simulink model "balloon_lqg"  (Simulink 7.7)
settings: Solver=ode45  StartTime=0.0  StopTime=50000  RelTol=1e-3
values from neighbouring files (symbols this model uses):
  Akf = A_balloon - Kkf * C_balloon    [design_KF_balloon.m]
  Bkf = [B_balloon Kkf]    [design_KF_balloon.m]
  C = V*rho_a*c_a    [balloon_init.m]
  Ckf = eye(3)    [design_KF_balloon.m]
  Dkf = zeros(3,4)    [design_KF_balloon.m]
  f = f / 10    [balloon_init.m]
  g = 9.80665    [balloon_init.m]
  m = input('Inserire le prime due cifre (esclusi zeri) del proprio numero di matricola:\n\n')    [balloon_init.m]
  rho_a = 1.2928    [balloon_init.m]
  Ta = 20+273.15    (= 293.15)    [balloon_init.m]
  theta_t = theta_t/50    [balloon_init.m]
  V = V*m*2    [balloon_init.m]
  x1_0 = x1_d    [balloon_init.m]
  x2_0 = 100    [balloon_init.m]
  x2_d = 120    [balloon_init.m]
  x3_0 = 0    [balloon_init.m]
  x3_d = 0    [balloon_init.m]
undefined symbols (not defined in the file or in its folder): K
libraries: simulink x3

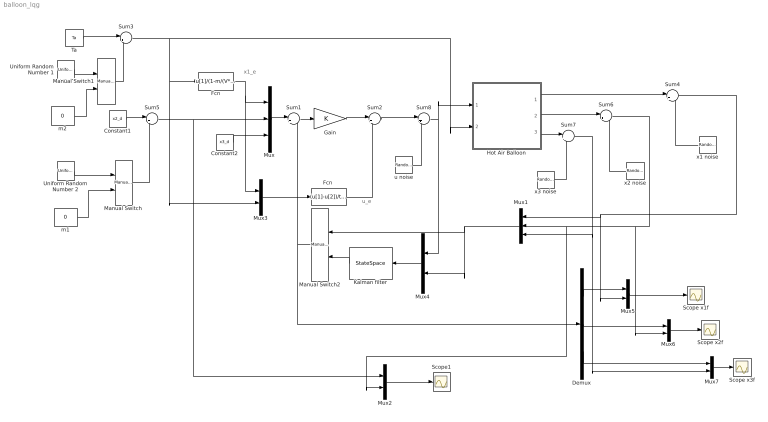
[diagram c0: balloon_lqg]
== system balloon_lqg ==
  note: x1_e
  note: u_e
  Constant1 : Constant  Value=x2_d
  Constant2 : Constant  Value=x3_d
  Demux : Demux  Outputs=3
  Fcn : Fcn  Expr=u[1]/(1-m/(V*rho_a))
  "Fcn " : Fcn  Expr=(u[1]-u[2])/theta_t
  Gain : Gain  Gain=K  Multiplication=Matrix(K*u)
  Hot Air Balloon : Subsystem  mask{V=V, m=m, C=C, theta_t=theta_t, f=f, g=g}
      mask prompts: V "Balloon's volume (V)"; m "Balloon's total mass (m)"; C "Thermal capacitance (C)"; theta_t "Thermal resistance (theta_t)"; f "Aerodynamic viscous friction (f)"; g "Gravitational acceleration (g)"
  Kalman filter : StateSpace  A=Akf  B=Bkf  C=Ckf  D=Dkf
  Manual Switch : simulink/Signal Routing/Manual Switch  SystemSampleTime=-1  sw=0  action=0  varsize=off
  Manual Switch1 : simulink/Signal Routing/Manual Switch  SystemSampleTime=-1  sw=0  action=0  varsize=off
  Manual Switch2 : simulink/Signal Routing/Manual Switch  SystemSampleTime=-1  sw=1  action=0  varsize=off
  Mux : Mux  Inputs=3
  Mux1 : Mux  Inputs=3
  Mux{2..7} (6 alike) : Mux  Inputs=2
  Scope x1f : Scope
  Scope x2f : Scope
  Scope x3f : Scope
  Scope1 : Scope
  Sum1 : Sum  Inputs=|+-
  Sum{2..8} (7 alike) : Sum  Inputs=|++
  Ta : Constant  Value=Ta
  Uniform Random Number 1 : UniformRandomNumber  SampleTime=200
  Uniform Random Number 2 : UniformRandomNumber  Minimum=-x2_d*0.1  Maximum=x2_d*0.1  Seed=1  SampleTime=1500
  m1 : Constant  Value=0
  m2 : Constant  Value=0
  u noise : RandomNumber  Variance=0.0001  Seed=4  SampleTime=0
  x1 noise : RandomNumber  Variance=0.00001  Seed=1  SampleTime=0
  x2 noise : RandomNumber  Variance=0.0005  Seed=2  SampleTime=0
  x3 noise : RandomNumber  Variance=0.0000005  Seed=3  SampleTime=0
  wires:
  Constant2/1 -> Mux/3
  Mux/1 -> Sum1/1
  Sum1/1 -> Gain/1
  Gain/1 -> Sum2/1
  "Fcn "/1 -> Sum2/2
  Mux1/1 -> Mux4/2, Manual Switch2/1
  Mux2/1 -> Scope1/1
  Ta/1 -> Sum3/1
  Constant1/1 -> Sum5/1
  Sum5/1 -> Mux/2, Mux2/1
  Sum3/1 -> Fcn/1, Mux3/2, Hot Air Balloon/2(Ta)
  Fcn/1 -> Mux/1, Mux3/1
  Mux3/1 -> "Fcn "/1
  Uniform Random Number 2/1 -> Manual Switch/1
  Manual Switch/1 -> Sum5/2
  m1/1 -> Manual Switch/2
  m2/1 -> Manual Switch1/2
  Manual Switch1/1 -> Sum3/2
  Uniform Random Number 1/1 -> Manual Switch1/1
  Hot Air Balloon/1(x1) -> Sum4/1
  Sum4/1 -> Mux1/1, Mux5/2
  Hot Air Balloon/2(x2) -> Sum6/1
  Sum6/1 -> Mux1/2, Mux2/2, Mux6/2
  Hot Air Balloon/3(x3) -> Sum7/1
  Sum7/1 -> Mux1/3, Mux7/2
  x1 noise/1 -> Sum4/2
  x2 noise/1 -> Sum6/2
  x3 noise/1 -> Sum7/2
  Sum2/1 -> Sum8/1
  Sum8/1 -> Hot Air Balloon/1(u), Mux4/1
  u noise/1 -> Sum8/2
  Mux4/1 -> Kalman filter/1
  Kalman filter/1 -> Manual Switch2/2
  Manual Switch2/1 -> Sum1/2, Demux/1
  Demux/1 -> Mux5/1
  Demux/2 -> Mux6/1
  Demux/3 -> Mux7/1
  Mux5/1 -> Scope x1f/1
  Mux6/1 -> Scope x2f/1
  Mux7/1 -> Scope x3f/1

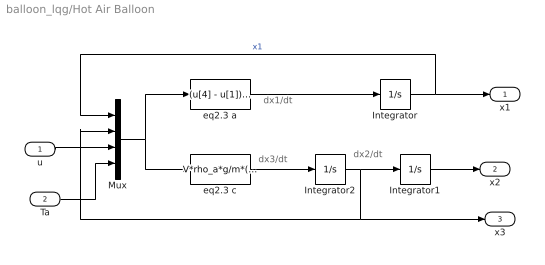
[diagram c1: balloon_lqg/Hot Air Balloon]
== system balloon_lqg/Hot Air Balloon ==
  note: dx2/dt
  note: dx3/dt
  note: dx1/dt
  u : Inport
  Ta : Inport  Port=2
  Integrator : Integrator  InitialCondition=x1_0
  Integrator1 : Integrator  InitialCondition=x2_0  LowerSaturationLimit=0
  Integrator2 : Integrator  InitialCondition=x3_0
  Mux : Mux
  eq2.3 a : Fcn  Expr=(u[4] - u[1])/(C*theta_t) + u[3]/C
  eq2.3 c : Fcn  Expr=V*rho_a*g/m*(1 - u[4]/u[1]) - f/m*u[2] - g
  x1 : Outport
  x2 : Outport  Port=2
  x3 : Outport  Port=3
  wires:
  Ta/1 -> Mux/4
  u/1 -> Mux/3
  Integrator1/1 -> x2/1
  Integrator2/1 -> Mux/2, x3/1, Integrator1/1
  Integrator/1 -> x1/1, Mux/1  "x1"
  Mux/1 -> eq2.3 c/1, eq2.3 a/1
  eq2.3 c/1 -> Integrator2/1
  eq2.3 a/1 -> Integrator/1
